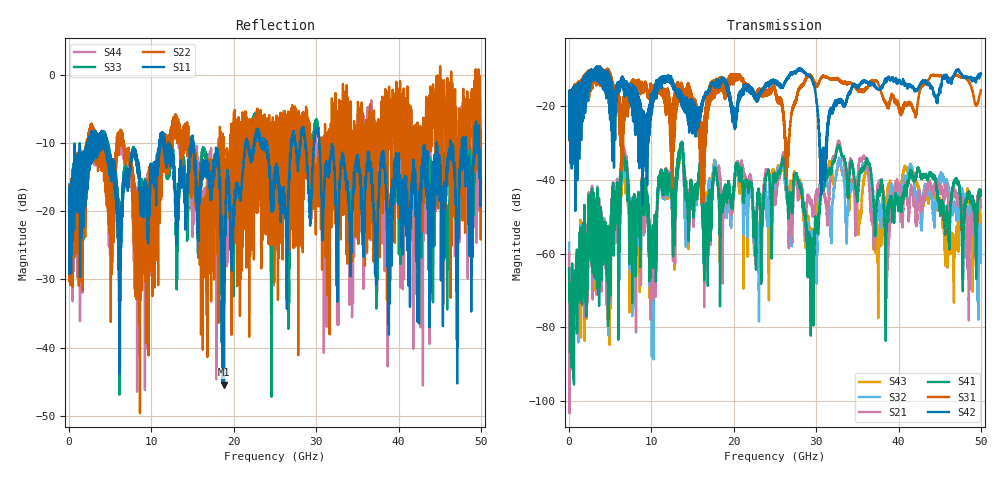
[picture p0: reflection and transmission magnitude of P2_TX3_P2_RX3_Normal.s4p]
!Keysight Technologies,N5225B,MY57041031,A.13.20.10
!Date: Friday, May 31, 2019 11:30:55
!Correction: S11(Full 4 Port(1,2,3,4))
!S12(Full 4 Port(1,2,3,4))
!S13(Full 4 Port(1,2,3,4))
!S14(Full 4 Port(1,2,3,4))
!S21(Full 4 Port(1,2,3,4))
!S22(Full 4 Port(1,2,3,4))
!S23(Full 4 Port(1,2,3,4))
!S24(Full 4 Port(1,2,3,4))
!S31(Full 4 Port(1,2,3,4))
!S32(Full 4 Port(1,2,3,4))
!S33(Full 4 Port(1,2,3,4))
!S34(Full 4 Port(1,2,3,4))
!S41(Full 4 Port(1,2,3,4))
!S42(Full 4 Port(1,2,3,4))
!S43(Full 4 Port(1,2,3,4))
!S44(Full 4 Port(1,2,3,4))
!S4P File: Measurements: <S11,S12,S13,S14>,
!<S21,S22,S23,S24>,
!<S31,S32,S33,S34>,
!<S41,S42,S43,S44>:
# Hz S  dB  R 50.0
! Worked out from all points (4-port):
!   5000 points, 10 MHz to 50 GHz, reference 50 ohm
!   strongest paths, dB at 10 MHz, 12.51 GHz, 25.01 GHz, 37.51 GHz, 50 GHz:
!     S42: -19.3, -14.2, -13.1, -15.3, -11.0
!     S31: -19.5, -42.1, -16.0, -13.6, -15.6
!     S41: -64.0, -40.5, -39.9, -44.0, -44.0
!     S21: -59.7, -40.6, -46.5, -40.9, -47.3
!     S32: -57.0, -43.1, -41.9, -45.5, -57.0
!     S43: -64.8, -42.4, -39.8, -62.5, -51.7
!   lowest |S11| = -45.4 dB at 18.81 GHz (marker M1), VSWR 1.01, Z = 50.5 - j0.241 ohm
!   |S11| at or under -10 dB: 4.63 GHz to 10.95 GHz (6.318 GHz wide, 81.1 % of centre); 15.04 GHz to 21.46 GHz (6.42 GHz wide, 35.2 % of centre); 30.38 GHz to 44.61 GHz (14.23 GHz wide, 37.9 % of centre)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
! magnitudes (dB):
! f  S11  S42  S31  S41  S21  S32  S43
! 10 MHz  -19.6  -19.3  -19.5  -64.0  -59.7  -57.0  -64.8
! 6.62 GHz  -15.9  -12.5  -19.8  -33.7  -31.6  -33.5  -36.3
! 10.07 GHz  -13.7  -21.5  -15.0  -57.7  -58.8  -71.1  -64.2
! 13.58 GHz  -12.6  -16.3  -13.6  -30.0  -29.9  -30.8  -31.1
! 18.81 GHz  -45.4  -12.3  -13.1  -44.3  -45.2  -45.6  -44.4
! 30.78 GHz  -20.8  -33.5  -11.7  -41.3  -42.2  -38.3  -36.8
! 50 GHz  -15.9  -11.0  -15.6  -44.0  -47.3  -57.0  -51.7
